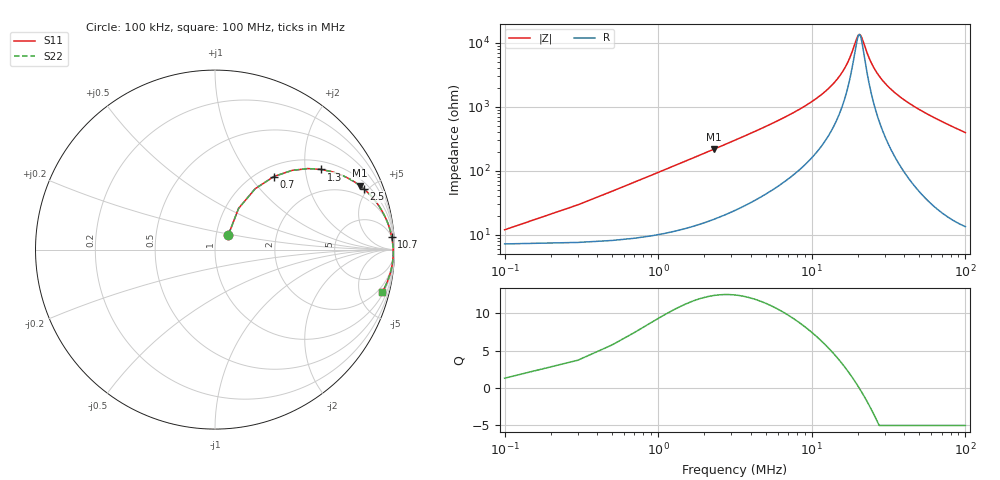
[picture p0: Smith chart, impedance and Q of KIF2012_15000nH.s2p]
!version-2
!date-12.2020
!Series
# MHz S RI R 50
!Freq ReS11 ImS11 ReS21 ImS21 ReS12 ImS12 ReS22 ImS22
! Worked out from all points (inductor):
!   501 points, 100 kHz to 100 MHz, reference 50 ohm
!   read as one part in series: L = 15 uH near 500 kHz
!   highest Q = 12.4 at 2.3 MHz (marker M1), where L = 15 uH
!   self-resonance near 20.3 MHz
!   S11 on the Smith chart (normalised r, x): 100 kHz: 1.14, +0.19; 700 kHz: 1.18, +1.32; 1.3 MHz: 1.23, +2.44; 2.5 MHz: 1.38, +4.72; 10.7 MHz: 5, +27; 100 MHz: 1.27, -7.91
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0.1  0.0747 0.0827  0.9253 -0.0827  0.9253 -0.0827  0.0747 0.0827
0.7  0.328 0.4071  0.672 -0.4071  0.672 -0.4071  0.328 0.4071
0.9  0.4286 0.4412  0.5714 -0.4412  0.5714 -0.4412  0.4286 0.4412
1.3  0.5921 0.4466  0.4079 -0.4466  0.4079 -0.4466  0.5921 0.4466
2.3  0.8065 0.3568  0.1935 -0.3568  0.1935 -0.3568  0.8065 0.3568
2.5  0.8295 0.3382  0.1705 -0.3382  0.1705 -0.3382  0.8295 0.3382
4.9  0.9432 0.1919  0.0568 -0.1919  0.0568 -0.1919  0.9432 0.1919
10.7  0.9843 0.0715  0.0157 -0.0715  0.0157 -0.0715  0.9843 0.0715
14.3  0.9897 0.0378  0.0103 -0.0378  0.0103 -0.0378  0.9897 0.0378
16.9  0.9915 0.0197  0.00848 -0.0197  0.00848 -0.0197  0.9915 0.0197
19.7  0.9925 0.00353  0.00749 -0.00353  0.00749 -0.00353  0.9925 0.00353
20.5  0.9927 -0.00066  0.00733 0.00066  0.00733 0.00066  0.9927 -0.00066
21.1  0.9928 -0.0037  0.00725 0.0037  0.00725 0.0037  0.9928 -0.0037
23.7  0.9929 -0.016  0.00711 0.016  0.00711 0.016  0.9929 -0.016
25.9  0.9927 -0.0256  0.00726 0.0256  0.00726 0.0256  0.9927 -0.0256
29.1  0.9922 -0.0384  0.00779 0.0384  0.00779 0.0384  0.9922 -0.0384
33.5  0.991 -0.0547  0.00904 0.0547  0.00904 0.0547  0.991 -0.0547
40.7  0.9879 -0.0788  0.0121 0.0788  0.0121 0.0788  0.9879 -0.0788
50.1  0.9825 -0.1075  0.0175 0.1075  0.0175 0.1075  0.9825 -0.1075
66.7  0.9695 -0.1535  0.0305 0.1535  0.0305 0.1535  0.9695 -0.1535
83.5  0.9527 -0.1957  0.0473 0.1957  0.0473 0.1957  0.9527 -0.1957
100  0.933 -0.2336  0.067 0.2336  0.067 0.2336  0.933 -0.2336
